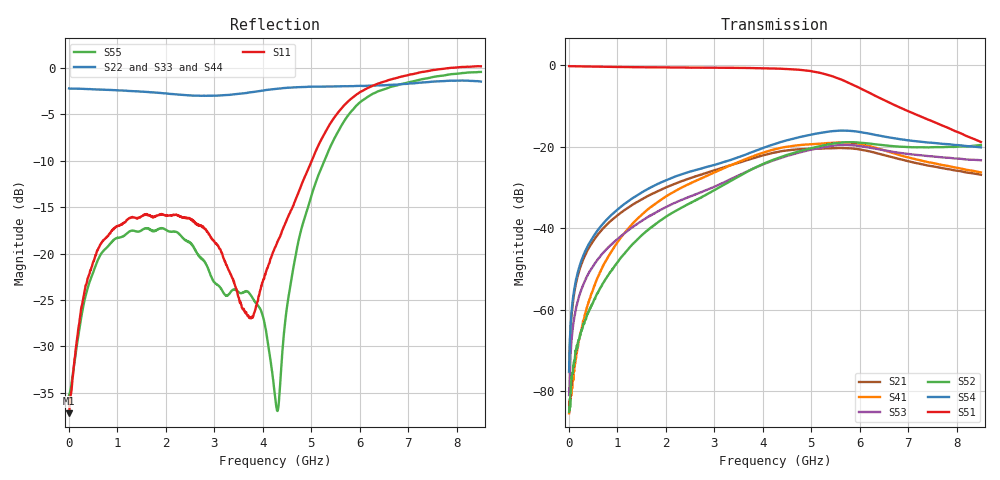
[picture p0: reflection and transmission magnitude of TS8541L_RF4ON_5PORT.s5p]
! Created with skrf (http://scikit-rf.org).
# Hz S RI R 50.0
!freq ReS11 ImS11 ReS12 ImS12 ReS13 ImS13
! ReS14 ImS14 ReS15 ImS15
! ReS21 ImS21 ReS22 ImS22 ReS23 ImS23
! ReS24 ImS24 ReS25 ImS25
! ReS31 ImS31 ReS32 ImS32 ReS33 ImS33
! ReS34 ImS34 ReS35 ImS35
! ReS41 ImS41 ReS42 ImS42 ReS43 ImS43
! ReS44 ImS44 ReS45 ImS45
! ReS51 ImS51 ReS52 ImS52 ReS53 ImS53
! ReS54 ImS54 ReS55 ImS55
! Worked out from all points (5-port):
!   1601 points, 10 MHz to 8.5 GHz, reference 50 ohm
!   strongest paths, dB at 10 MHz, 2.132 GHz, 4.255 GHz, 6.378 GHz, 8.5 GHz:
!     S51: -0.2, -0.5, -0.7, -7.8, -18.8
!     S54: -75.2, -27.6, -19.3, -17.2, -20.1
!     S52: -85.1, -36.2, -23.0, -19.4, -19.5
!     S53: -81.0, -34.1, -23.2, -20.6, -23.3
!     S41: -85.4, -31.3, -20.6, -20.4, -26.3
!     S21: -75.3, -29.3, -21.4, -21.6, -26.8
!   lowest |S11| = -37.2 dB at 10 MHz (marker M1), VSWR 1.03, Z = 51.4 - j0.0906 ohm
!   |S11| at or under -10 dB: start of sweep to 5.013 GHz
